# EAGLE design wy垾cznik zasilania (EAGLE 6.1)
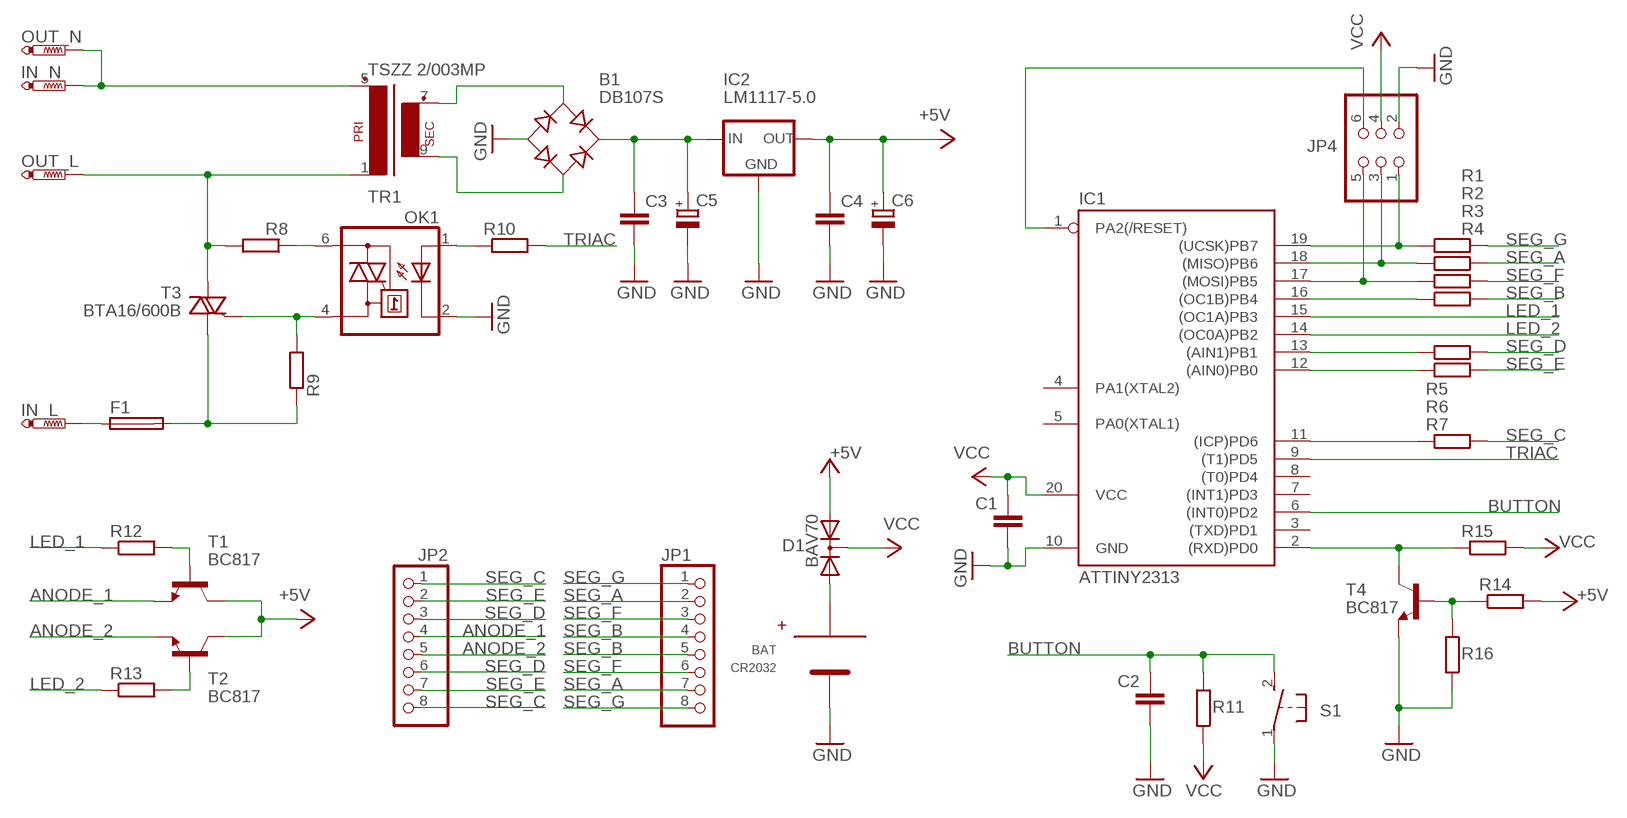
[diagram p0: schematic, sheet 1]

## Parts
B1  DB107S  DBLS201G  [DBS]
BAT  CR2032  [HOLDER-CR2032]
C1  C-EUC0805  [C0805]
C2  C-EUC0805  [C0805]
C3  C-EUC0805  [C0805]
C4  C-EUC0805  [C0805]
C5  CPOL-EUE2.5-7  [E2,5-7]
C6  CPOL-EUE2.5-7  [E2,5-7]
D1  BAV70  DIODE-2AC|CASOT23  [SOT23]
F1  SH22,5  [SH22,5]
IC1  ATTINY2313  TINY2313-*S*  [SO20L$]
IC2  LM1117-5.0  LM1117TO252  [TO252]
IN_L  PTR1PAD1-17Y  [P1-17Y]
IN_N  PTR1PAD1-17Y  [P1-17Y]
JP1  PINHD-1X8  [1X08]
JP2  PINHD-1X8  [1X08]
JP4  PINHD-2X3  [2X03]
OK1  MOC3033M  [DIL06]
OUT_L  PTR1PAD1-17Y  [P1-17Y]
OUT_N  PTR1PAD1-17Y  [P1-17Y]
R1  R-EU_R0805  [R0805]
R2  R-EU_R0805  [R0805]
R3  R-EU_R0805  [R0805]
R4  R-EU_R0805  [R0805]
R5  R-EU_R0805  [R0805]
R6  R-EU_R0805  [R0805]
R7  R-EU_R0805  [R0805]
R8  R-EU_0411/3V  [0411V]
R9  R-EU_0414/5V  [0414V]
R10  R-EU_R0805  [R0805]
R11  R-EU_R0805  [R0805]
R12  R-EU_R0805  [R0805]
R13  R-EU_R0805  [R0805]
R14  R-EU_R0805  [R0805]
R15  R-EU_R0805  [R0805]
R16  R-EU_R0805  [R0805]
S1  31-XX  [B3F-31XX]
T1  BC817  BC817-40-NPN-SOT23-BEC  [SOT23-BEC]
T2  BC817  BC817-40-NPN-SOT23-BEC  [SOT23-BEC]
T3  BTA16/600B  BT138-V  [TO220BV]
T4  BC817  BC817-40-NPN-SOT23-BEC  [SOT23-BEC]
TR1  TSZZ 2/003MP  EI30-1  [EI30-1]

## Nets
+5V: C4.1 C6.+ D1.1(A1) IC2.3(OUT) R14.2 T1.C T2.C
ANODE_1: JP2.4 T1.E
ANODE_2: JP2.5 T2.E
BUTTON: C2.1 IC1.6((INT0)PD2) R11.2 S1.2(S)
GND: B1.- BAT.1(-) C1.2 C2.2 C3.2 C4.2 C5.- C6.- IC1.10(GND) IC2.1(GND) JP4.2 OK1.2(C) R16.1 S1.1(P) T4.E
LED_1: IC1.15((OC1A)PB3) R12.1
LED_2: IC1.14((OC0A)PB2) R13.1
N$1: IN_N.TP OUT_N.TP TR1.5(P2)
N$2: OUT_L.TP R8.2 T3.T2(A2) TR1.1
N$3: F1.1 IN_L.TP
N$4: IC1.19((UCSK)PB7) JP4.1 R1.1
N$5: R12.2 T1.B
N$6: IC1.18((MISO)PB6) JP4.3 R2.1
N$7: IC1.17((MOSI)PB5) JP4.5 R3.1
N$8: IC1.16((OC1B)PB4) R4.1
N$9: IC1.11((ICP)PD6) R7.1
N$10: IC1.12((AIN0)PB0) R6.1
N$11: IC1.13((AIN1)PB1) R5.1
N$12: OK1.6(A2) R8.1
N$13: OK1.4(A1) R9.2 T3.G
N$14: F1.2 R9.1 T3.T1(A1)
N$15: B1.AC1 TR1.7(S3)
N$16: IC1.1(PA2(/RESET)) JP4.6
N$17: B1.AC2 TR1.9(S4)
N$18: B1.+ C3.1 C5.+ IC2.2(IN)
N$19: R13.2 T2.B
N$21: IC1.2((RXD)PD0) R15.1 T4.C
N$22: R14.1 R16.2 T4.B
N$23: BAT.2(+) D1.2(A2)
N$24: OK1.1(A) R10.1
SEG_A: JP1.2 JP1.7 R2.2
SEG_B: JP1.4 JP1.5 R4.2
SEG_C: JP2.1 JP2.8 R7.2
SEG_D: JP2.3 JP2.6 R5.2
SEG_E: JP2.2 JP2.7 R6.2
SEG_F: JP1.3 JP1.6 R3.2
SEG_G: JP1.1 JP1.8 R1.2
TRIAC: IC1.9((T1)PD5) R10.2
VCC: C1.1 D1.3(C) IC1.20(VCC) JP4.4 R11.1 R15.2
Unconnected: IC1.3((TXD)PD1) IC1.4(PA1(XTAL2)) IC1.5(PA0(XTAL1)) IC1.7((INT1)PD3) IC1.8((T0)PD4)

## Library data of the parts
B1 = rectifier:DB?*G: Single Phase 1.0 AMP Glass Passivated Bridge Rectifier Taiwan Semiconductor Co.,Ltd. - TSC Source: http://www.taiwansemi.com/TSCbig5/ezcatfiles/cust/img/img/db101g.pdf http://www.ts.com.tw/db/pictures/modules/PDT/PDT060207001/DBLS201G.pdf
BAT = CR2032-holder:CR2032
C1-C4 = rcl:C-EU: CAPACITOR, European symbol
C5 C6 = rcl:CPOL-EU: POLARIZED CAPACITOR, European symbol
D1 = diode:DIODE-2AC|CA: Dual DIODE Anode-Cathode|Cathode-Anode
F1 = fuse:SH22,5: FUSE HOLDER; MF: SCHURTER; MPN: 0031.8201; OC_FARNELL: 1162740; OC_NEWARK: 96F8317
IC1 = avr-6:TINY2313*: Atmel Tiny2313 2K Flash, 128 bytes EEPROM, 128 bytes RAM
IC2 = v-reg-2:LM1117
IN_L IN_N OUT_L OUT_N = testpad:PTR1: TEST PIN
JP1 JP2 = pinhead:PINHD-1X8: PIN HEADER
JP4 = pinhead:PINHD-2X3: PIN HEADER
OK1 = optocoupler:MOC30*: 6-Pin DIP Zero-Cross Optoisolators Triac Driver Output (250/400 Volt Peak) Source: http://www.fairchildsemi.com/ds/MO/MOC3043-M.pdf; MF: FAIRCHILD SEMICONDUCTOR; MPN: MOC3033-M; OC_FARNELL: 1133987; OC_NEWARK: 72K8898
R1-R16 = rcl:R-EU_: RESISTOR, European symbol
S1 = switch-omron:31-XX: OMRON SWITCH; MPN: B3F-3100; OC_FARNELL: 959704; OC_NEWARK: 36M3582
T1 T2 T4 = transistor:*-NPN-: NPN Transistror BF959 corrected 2008.03.06
T3 = triac:BT138: TRIAC Source: http://www.semiconductors.philips.com BT138_SERIES_2.pdf
TR1 = trafo:EI30-1: TRANSFORMER 1 primary winding, 1 secondary winding ERA

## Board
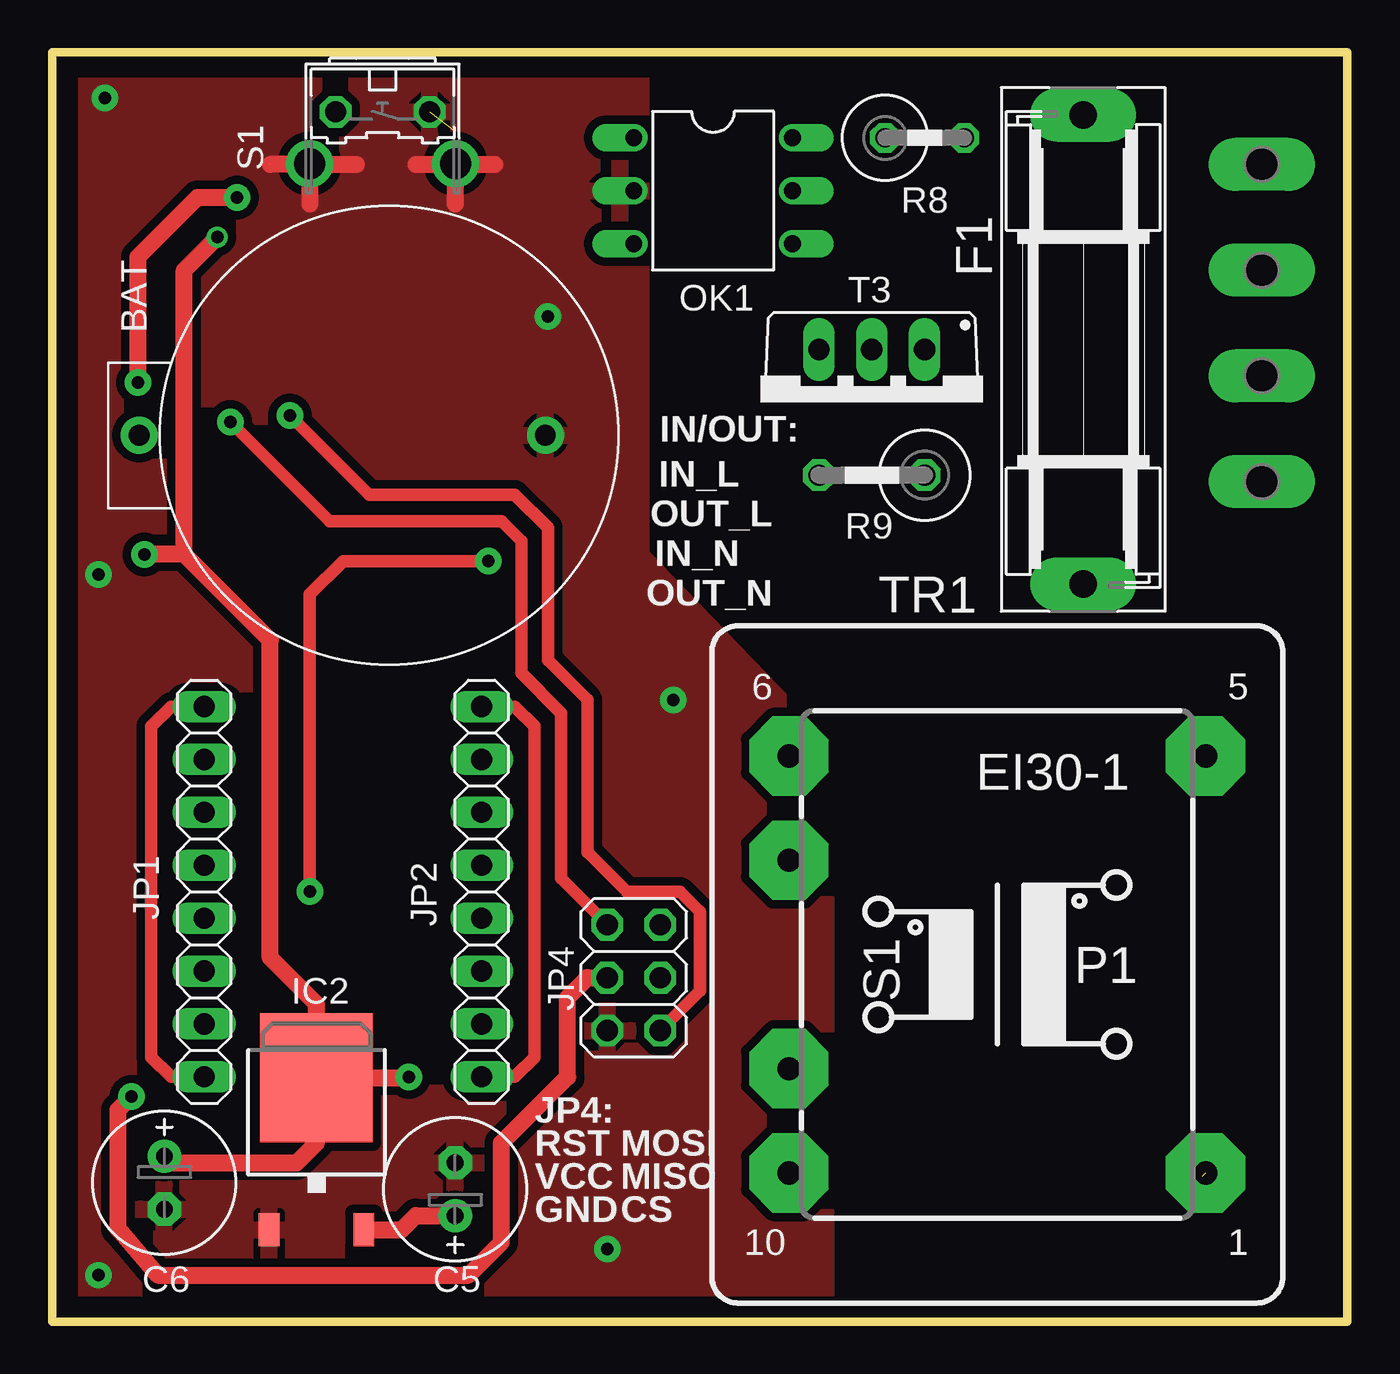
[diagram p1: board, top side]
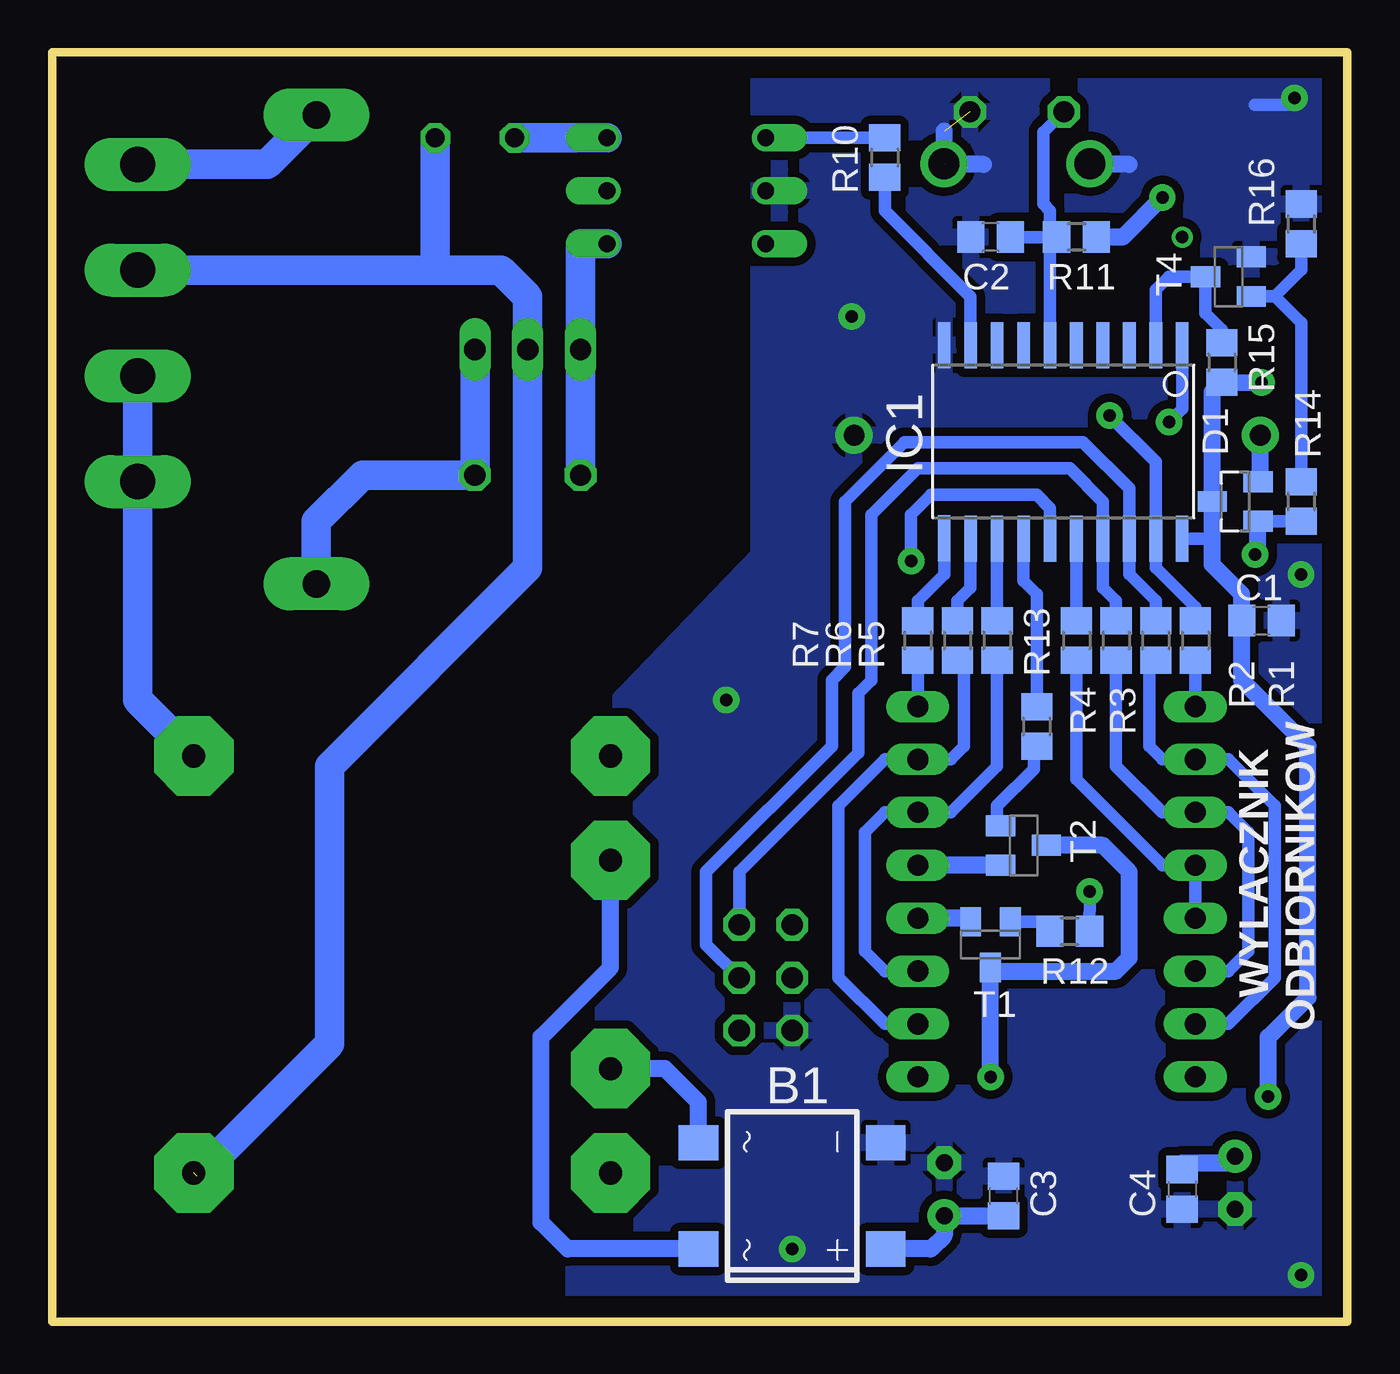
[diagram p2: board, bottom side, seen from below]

Size 62.22 x 60.95 mm. Coordinates in mm from the lower left corner, seen from the top.
Outline: 0,0 62.22,0 62.22,60.95 0,60.95 0,0
Copper layers (1*16): Top 0.035mm / dielectric 1.5mm / Bottom 0.035mm
Design rules: minimum track width 10mil, minimum drill 24mil, track to track 8mil, track to pad 8mil, pad to pad 8mil, via to via 8mil, smd to smd 8mil, copper to edge 40mil, drill to drill 8mil, minimum pad ring 10mil, minimum via ring 8mil, stop-mask expansion 4mil, vias tented up to drill 0mil, thermal gap 10mil

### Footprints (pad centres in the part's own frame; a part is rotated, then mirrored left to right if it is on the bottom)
DBS = smd 1.7 x 1.9: + -2.55,-4.5; - 2.55,-4.5; AC1 -2.55,4.5; AC2 2.55,4.5
HOLDER-CR2032 = drill 1 pad 1.778: 1 0,-7.5; 2 0,12
C0805 = smd 1.3 x 1.5: 1 -0.95,0; 2 0.95,0
E2,5-7 = drill 0.813 pad 1.6: + -1.27,0 | drill 0.813 pad 1.6 octagon: - 1.27,0
SOT23 = smd 1 x 1.4: 1 -0.95,-1.1; 2 0.95,-1.1; 3 0,1.1
SH22,5 = drill 1.321 pad 2.54 long: 1 -11.252,0; 2 11.252,0
SO20L$ = smd 0.61 x 2.21: 1 -5.715,-4.636; 2 -4.445,-4.636; 3 -3.175,-4.636; 4 -1.905,-4.636; 5 -0.635,-4.636; 6 0.635,-4.636; 7 1.905,-4.636; 8 3.175,-4.636; 9 4.445,-4.636; 10 5.715,-4.636; 11 5.715,4.61; 12 4.445,4.636; 13 3.175,4.636; 14 1.905,4.636; 15 0.635,4.636; 16 -0.635,4.636; 17 -1.905,4.636; 18 -3.175,4.636; 19 -4.445,4.636; 20 -5.715,4.636
TO252 = smd 1 x 1.6: 1 -2.28,-6.07; 2 2.28,-6.07 | smd 5.4 x 6.2: 3 0,1.23
P1-17Y = drill 1.702 pad 2.121 long: TP 0,0
1X08 = drill 1.016 long: 1 -8.89,0; 2 -6.35,0; 3 -3.81,0; 4 -1.27,0; 5 1.27,0; 6 3.81,0; 7 6.35,0; 8 8.89,0
2X03 = drill 1.016 octagon: 1 -2.54,-1.27; 2 -2.54,1.27; 3 0,-1.27; 4 0,1.27; 5 2.54,-1.27; 6 2.54,1.27
DIL06 = drill 0.813 offset: 1 -2.54,-3.81; 2 0,-3.81; 3 2.54,-3.81; 4 2.54,3.81; 5 0,3.81; 6 -2.54,3.81
R0805 = smd 1.3 x 1.5: 1 -0.95,0; 2 0.95,0
0411V = drill 0.914 octagon: 1 -2.54,0; 2 1.27,0
0414V = drill 1.016 octagon: 1 -2.54,0; 2 2.54,0
B3F-31XX = drill 1.016 octagon: 1 -2.261,-1.245; 2 2.261,-1.245 | drill 1.499 pad 2.159: 3 -3.505,1.245; 4 3.505,1.245
SOT23-BEC = smd 1 x 1.4: B -0.95,-1.1; C 0,1.1; E 0.95,-1.1
TO220BV = drill 1.016 long: G 2.54,-2.54; T1 -2.54,-2.54; T2 0,-2.54
EI30-1 = drill 1.118 pad 3.81 octagon: 1 -10.008,10.008; 5 -10.008,-10.008; 6 10.008,-10.008; 7 10.008,-5.004; 9 10.008,5.004; 10 10.008,10.008

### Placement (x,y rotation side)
B1  26.67,6.03 90 bottom
BAT  16.19,42.55 90 top
C1  4.13,33.66 0 bottom
C2  17.14,52.07 180 bottom
C3  16.51,6.03 90 bottom
C4  7.94,6.35 270 bottom
C5  19.37,6.35 90 top
C6  5.4,6.67 270 top
D1  5.4,39.37 90 bottom
F1  49.53,46.67 270 top
IC1  13.65,42.23 180 bottom
IC2  12.7,10.48 0 top
IN_L  58.1,55.56 90 top
IN_N  58.1,45.4 90 top
JP1  7.3,20.64 90 top
JP2  20.64,20.64 90 top
JP4  27.94,16.51 90 top
OK1  31.75,54.29 270 top
OUT_L  58.1,50.48 90 top
OUT_N  58.1,40.32 90 top
R1  7.3,32.7 270 bottom
R2  9.21,32.7 270 bottom
R3  11.11,32.7 270 bottom
R4  13.02,32.7 270 bottom
R5  16.83,32.7 270 bottom
R6  18.73,32.7 270 bottom
R7  20.64,32.7 270 bottom
R8  42.55,56.83 0 top
R9  39.37,40.64 180 top
R10  22.23,55.88 270 bottom
R11  13.02,52.07 180 bottom
R12  13.34,18.73 180 bottom
R13  14.92,28.57 270 bottom
R14  2.22,39.37 270 bottom
R15  6.03,46.04 270 bottom
R16  2.22,52.7 270 bottom
S1  15.88,56.83 180 top
T1  17.14,18.1 180 bottom
T2  15.56,22.86 270 bottom
T3  39.37,44.13 180 top
T4  5.71,50.16 90 bottom
TR1  45.4,17.14 180 top

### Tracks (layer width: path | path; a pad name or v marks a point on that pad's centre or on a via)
+5V  (via drill 0.6, 0.6 pad 1.27)
  Top 0.813: v7.94,52.07 6.35,50.48 6.35,36.83 | 6.35,36.83 v4.45,36.83 | 6.35,36.83 10.48,32.7 10.48,17.46 12.7,15.24 IC2.3 | IC2.3 17.11,11.71 v17.14,11.75 | IC2.3 12.7,8.57 11.75,7.62 5.4,7.62 C6.+
  Bottom 0.61: D1.1 R14.2
  Bottom 0.813: D1.1 4.3,36.98 v4.45,36.83 | T2.C 11.75,22.86 10.48,21.59 10.48,17.46 11.11,16.83 17.14,16.83 T1.C v17.14,11.75 | C4.1 7.94,7.62 5.39,7.62 5.4,7.62 C6.+
ANODE_1
  Bottom 0.61: T1.E 18.1,19.05
  Bottom 0.813: JP2.4 18.09,19.37 T1.E
ANODE_2
  Bottom 0.813: JP2.5 T2.E
BUTTON
  Bottom 0.61: R11.2 C2.1 | S1.2 14.6,57.09 14.61,53.66 14.29,53.34 14.29,52.39 R11.2 | IC1.6 14.29,52.07 R11.2
GND  (via drill 0.6 pad 1.27)  (3 unrouted)
  Top 0.813: 12.38,55.56 10.48,55.56 | 12.38,55.56 14.61,55.56 | 12.38,55.56 12.38,53.66 | 17.46,55.56 19.37,55.56 | 19.37,55.56 21.27,55.56 | 19.37,55.56 19.37,53.66
  Bottom 0.61: 2.85,58.42 4.45,58.42
  Bottom 0.813: 10.48,55.56 12.38,55.56 | 19.37,57.15 19.37,55.56 17.46,55.56
  other vias: 29.84,29.84 2.54,58.74 2.22,2.22 26.67,3.49 23.81,48.26 2.22,35.88
  pour Bottom (isolate 0.406): -1.59,-0.64 37.15,-0.64 37.15,27.62 28.26,36.83 28.26,61.59 -1.59,61.59
  pour Top (isolate 0.406): -0.64,61.59 28.26,61.59 28.26,36.83 37.15,27.62 37.15,-1.59 -0.64,-1.27
LED_1  (via drill 0.6 pad 1.27)
  Top 0.61: v12.38,20.64 12.38,34.92 13.97,36.51 v20.95,36.51
  Bottom 0.61: IC1.15 14.29,39.05 14.92,39.69 20,39.69 20.95,38.73 v20.95,36.51 | R12.1 v12.38,20.64
LED_2
  Bottom 0.61: IC1.14 15.56,35.56 14.92,34.92 R13.1
N$1
  Bottom 1.422: TR1.5 58.1,29.84 OUT_N.TP IN_N.TP
N$2  (1 unrouted)
  Bottom 1.422: 43.81,50.48 40.64,50.48 39.37,49.21 T3.T2 39.37,36.2 48.9,26.67 48.9,13.34 55.24,6.99 | 43.81,50.48 OUT_L.TP | 43.81,50.48 R8.2
N$3
  Bottom 1.422: F1.1 51.89,55.56 IN_L.TP
N$4  (via drill 0.6 pad 1.27)
  Top 0.61: v11.43,43.5 15.24,39.69 22.23,39.69 23.81,38.1 23.81,31.75 25.72,29.84 25.72,22.54 27.62,20.64 30.16,20.64 31.11,19.68 31.11,15.88 JP4.1
  Bottom 0.61: R1.1 7.3,34.29 9.21,36.2 IC1.19 9.21,41.27 v11.43,43.5
N$5
  Bottom 0.61: T1.B 13.97,19.2 R12.2
N$6
  Bottom 0.61: R2.1 9.21,34.61 10.48,35.88 IC1.18 10.48,40.01 12.7,42.23 21.27,42.23 24.13,39.37 24.13,31.43 24.77,30.8 24.77,27.62 30.8,21.59 30.8,18.1 JP4.3
N$7
  Bottom 0.61: R3.1 11.11,34.61 11.75,35.24 IC1.17 11.75,39.37 13.34,40.96 20.64,40.96 22.86,38.73 22.86,30.8 23.5,30.16 23.5,27.3 29.21,21.59 JP4.5
N$8
  Bottom 0.61: R4.1 IC1.16
N$9
  Bottom 0.61: R7.1 20.64,34.61 19.37,35.88 IC1.11
N$10
  Bottom 0.61: R6.1 18.73,34.61 18.1,35.24 IC1.12
N$11
  Bottom 0.61: R5.1 IC1.13
N$12
  Bottom 1.422: OK1.6 R8.1
N$13
  Bottom 1.422: OK1.4 36.83,51.75 T3.G R9.2
N$14
  Bottom 1.422: T3.T1 R9.1 47.31,40.64 49.53,38.42 F1.2
N$15
  Bottom 0.813: B1.AC1 37.45,3.48 38.73,4.76 38.73,13.65 35.4,16.99 TR1.7
N$16  (via drill 0.6 pad 1.27)
  Top 0.61: v8.57,43.18 13.34,38.42 21.59,38.42 22.54,37.47 22.54,31.11 24.45,29.21 24.45,21.27 JP4.6
  Bottom 0.61: IC1.1 7.94,43.81 v8.57,43.18
N$17
  Bottom 0.813: TR1.9 32.78,12.14 31.17,10.53 B1.AC2
N$18
  Top 0.813: IC2.2 16.79,4.41 17.46,5.08 C5.+
  Bottom 0.813: B1.+ 20.01,3.48 19.37,4.13 C5.+ C3.1
N$19
  Bottom 0.61: R13.2 15.07,27.62 15.07,26.52 16.83,24.77 16.83,23.81 T2.B
N$21
  Bottom 0.61: R15.1 6.03,47.62 6.82,48.41 T4.C 8.57,50.16 9.21,49.53 IC1.2
N$22
  Bottom 0.61: R14.1 2.22,47.94 3.5,49.22 | 3.5,49.22 T4.B | R16.2 2.22,50.49 3.5,49.22
N$23
  Bottom 0.813: BAT.2 4.19,40.42 D1.2
N$24
  Bottom 0.61: R10.1 OK1.1
SEG_A
  Bottom 0.61: JP1.2 5.71,14.29 3.49,16.51 3.49,24.77 5.71,26.99 JP1.7 8.89,26.99 9.53,27.62 9.53,31.75 9.52,31.75 R2.2
SEG_B
  Bottom 0.61: JP1.4 JP1.5 8.89,21.91 13.02,26.04 R4.2
SEG_C
  Top 0.61: JP2.8 22.23,29.53 23.18,28.57 23.18,12.7 22.23,11.75 JP2.1
  Bottom 0.61: JP2.8 R7.2
SEG_D
  Bottom 0.61: JP2.3 22.23,16.83 23.18,17.78 23.18,23.5 22.23,24.45 JP2.6 19.05,24.45 16.83,26.67 R5.2
SEG_E
  Bottom 0.61: JP2.2 22.23,14.29 24.45,16.51 24.45,24.77 22.23,26.99 JP2.7 19.05,26.99 18.41,27.62 18.41,31.75 R6.2
SEG_F
  Bottom 0.61: JP1.3 5.71,16.83 4.76,17.78 4.76,23.5 5.71,24.45 JP1.6 8.89,24.45 11.11,26.67 R3.2
SEG_G
  Top 0.61: JP1.8 5.71,29.53 4.76,28.57 4.76,12.7 5.71,11.75 JP1.1
  Bottom 0.61: JP1.8 R1.2
TRIAC
  Bottom 0.61: IC1.9 18.1,49.21 22.23,53.34 R10.2
VCC  (via drill 0.6 pad 1.27)
  Top 0.813: JP4.4 25.72,16.51 24.77,15.56 24.77,11.75 21.59,8.57 21.59,3.81 20,2.22 5.08,2.22 3.17,4.45 3.17,10.16 v3.81,10.79 | v4.13,45.09 4.13,51.12 6.99,53.98 v8.89,53.98
  Bottom 0.61: IC1.20 6.69,37.59 6.5,37.78
  Bottom 0.813: v3.81,10.79 3.81,13.65 1.91,15.56 1.91,27.62 5.08,30.8 C1.1 5.08,34.92 6.5,36.34 6.5,37.78 D1.3 6.5,44.62 R15.2 v4.13,45.09 | v8.89,53.98 10.79,52.07 R11.1

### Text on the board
tNames: IN/OUT: | JP4: | RST | MOSI | VCC | MISO | GND | CS
bNames: WYLACZNIK | ODBIORNIKOW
